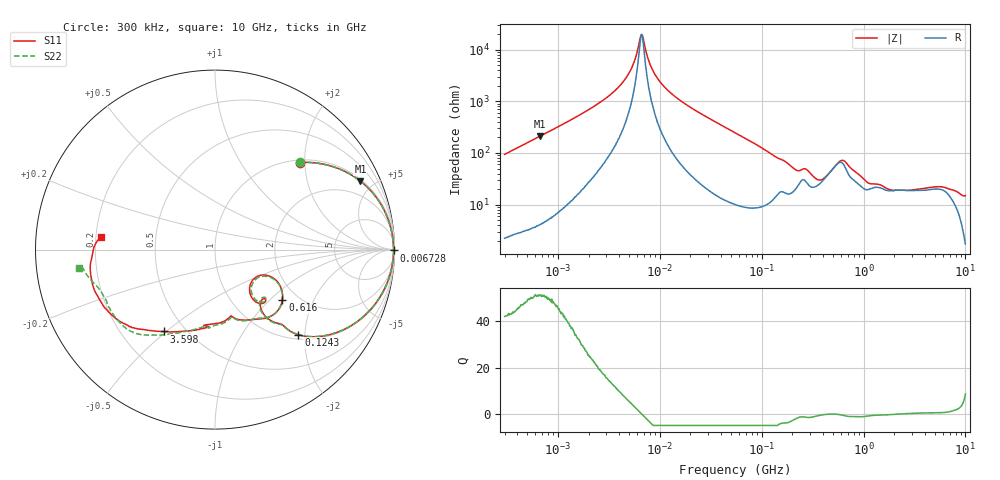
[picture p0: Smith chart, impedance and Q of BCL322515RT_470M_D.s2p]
! S-Parameter Data Generated by TDK Corporation
! Copyright(C) 2024 TDK Corporation.
! All Rights Reserved.
! TDK P/N: BCL322515RT-470M-D (SMD / SMT Inductor (Coil))
! Property: L=47uH at 1MHz
! Size(LxWxT): 3.2x2.5x1.5mm
! Model Type: s2p (Touchstone File Format Version 1.0)
! Frequency: DC=Yes Start=0.3MHz Stop=10000MHz 802points Log-sweep
! Model Generated on May 28, 2024
! Terms and conditions regarding TDK Simulation Models:
! 1)This simulation model is being provided solely for informational
!  purposes. Please refer to the specifications of the products in
!  terms of detailed characteristics of such products.
! 2)In no event shall TDK Corporation of any of its subsidiaries be
!  liable for any loss or damage arising, directly or indirectly,
!  from any information contained in this simulation model, including,
!  but not limited to loss or damages arising from any inaccuracies,
!  omissions or errors in connection with such information.
! 3)Any and all copyrights on this simulation model are owned by
!  TDK Corporation.  Duplication or redistribution of this simulation
!  model without prior written permission from TDK Corporation
!  is prohibited.
! 4)This simulation model is subject to any modification or change
!  without any prior notice.
! 5)Neither TDK Corporation nor any of its subsidiaries shall make any
!  warranty, express or implied, including but not limited to the
!  correctness, implied warranties of merchantability and fitness for
!  a particular purpose with respect to this simulation models.
! 6)The use of this simulation model shall be deemed to have consented
!  to the terms and conditions hereof.
! Port Assignments:
!  1 ---@@@--- 2
! Applicable Conditions:
!  Temperature = 25 degC
!  DC Bias Current = 0 A
!  Small Signal Operation
# Hz S MA R 50
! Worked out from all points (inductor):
!   801 points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, 300 kHz to 10 GHz, reference 50 ohm
!   read as one part in series: L = 49.8 uH near 318.3 kHz
!   highest Q = 51.3 at 663.1 kHz (marker M1), where L = 50.3 uH
!   self-resonance near 6.556 MHz
!   S11 on the Smith chart (normalised r, x): 300 kHz: 1.05, +1.88; 6.728 MHz: open; 124.3 MHz: 1.09, -1.85; 616 MHz: 1.66, -1.20; 3.598 GHz: 0.38, -0.49; 10 GHz: 0.22, +0.05
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300000  0.6764 45.8  0.7202 -42.8  0.7204 -42.7  0.6765 45.8
663069  0.8956 25.2  0.4275 -63.7  0.4276 -63.7  0.8955 25.2
1713600  0.9795 9.8  0.1709 -78.3  0.171 -78.3  0.9796 9.8
4363314  0.994 2.2  0.04202 -80.7  0.04202 -80.6  0.9939 2.2
5354396  0.9947 1.0  0.02152 -75.3  0.02153 -75.3  0.9947 1.0
6384737  0.9949 0.0  0.00627 -37.8  0.006304 -37.2  0.9951 0.0
6727812  0.9949 -0.3  0.005148 14.1  0.00516 14.1  0.9951 -0.3
7771787  0.9949 -1.1  0.01608 71.0  0.01607 70.6  0.9949 -1.1
9671944  0.9942 -2.4  0.03759 79.8  0.0376 79.9  0.9943 -2.4
1.763281e7  0.988 -6.8  0.1098 80.1  0.1099 80.1  0.988 -6.8
5.477226e7  0.9155 -23.1  0.367 64.6  0.3671 64.6  0.9156 -23.1
1.242712e8  0.6641 -45.6  0.6735 37.7  0.6737 37.8  0.6652 -45.5
2.039737e8  0.4367 -52.8  0.773 18.5  0.7733 18.6  0.4337 -53.2
3.126428e8  0.3432 -52.6  0.7826 8.5  0.7829 8.5  0.347 -51.2
4.089972e8  0.2732 -35.2  0.7516 -3.1  0.7518 -3.0  0.2819 -35.4
6.15965e8  0.4694 -36.9  0.5777 -1.1  0.5779 -1.1  0.4713 -37.4
1.024756e9  0.4029 -73.1  0.7623 -6.0  0.7625 -6.0  0.4101 -72.6
1.767019e9  0.4147 -92.5  0.7503 -24.0  0.7505 -24.0  0.422 -90.0
3.598403e9  0.5382 -122.0  0.6383 -54.1  0.6386 -54.1  0.5456 -119.8
6.576072e9  0.6721 -145.0  0.478 -82.5  0.4778 -82.6  0.6707 -144.9
8.322921e9  0.707 -167.4  0.4136 -102.2  0.414 -102.3  0.696 -163.9
1e10  0.6364 173.6  0.3243 -113.5  0.3241 -113.6  0.7644 -172.3
